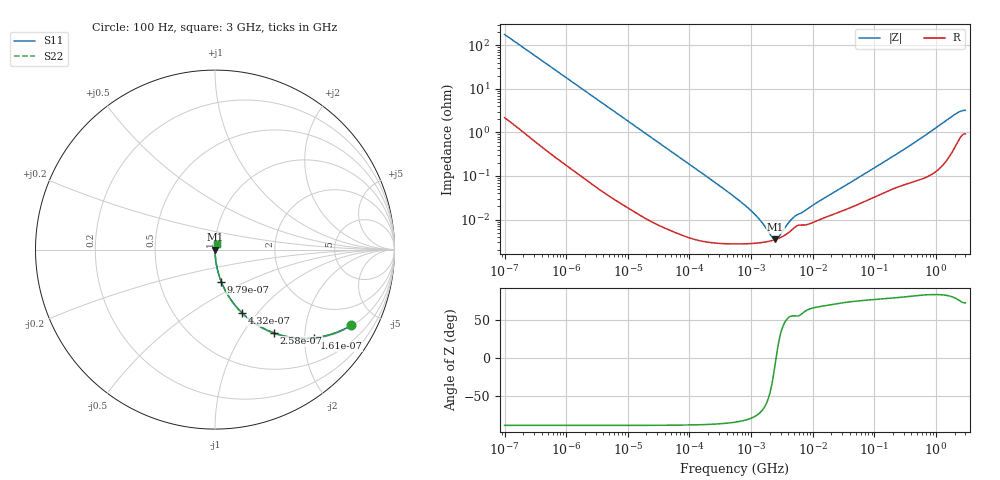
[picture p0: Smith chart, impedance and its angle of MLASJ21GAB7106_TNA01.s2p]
! MLASJ21GAB7106_TNA01  S-PARAMETER MODEL  ( Standard Model )
! Model Generated by TAIYO YUDEN Corporation (http://www.ty-top.com)
! Version 1.0
! TAIYO YUDEN Control No. 220601
! Copyright(c) 2009 TAIYO YUDEN CO.,LTD. All Rights Reserved.
! Product Description (link to TY-COMPAS)
! https://ds.yuden.co.jp/TYCOMPAS/or/detail?pn=MLASJ21GAB7106KTNA01&u=M
! Products Name : Multilayer Ceramic Capacitors
! Characteristics :
!  Capacitance : 10 [uF] , Rated Voltage : 6.3 [V] , TCC : X7R
!  Case Size : 2.0 x 1.25 / 0.079 x 0.049 [mm/inch] , Thickness : 1.25 / 0.049 [mm/inch]
!  (Conditions: Temperature = 25 [degC] , DC Bias Voltage = 0 [V])
! External Node Assignments :
!  1  o---| |---o  2
! GND o---------o GND
! Frequency Range : 100Hz  -  3GHz  [ 401 STEP ]
# MHZ S RI R 50
! Freq[MHz].  S11 Real  S11 Imag  S21 Real  S21 Imag  S12 Real  S12 Imag  S22 Real  S22 Imag
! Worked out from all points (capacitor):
!   401 points, 100 Hz to 3 GHz, reference 50 ohm
!   read as one part in series: C = 8.92 uF near 109 Hz
!   lowest |Z| = 3.49 mohm at 2.471 MHz (marker M1)
!   series resonance near 2.541 MHz, so ESL is about 440 pH
!   S11 on the Smith chart (normalised r, x): 100 Hz: 1.04, -3.56; 161 Hz: 1.03, -2.23; 258 Hz: 1.02, -1.39; 432 Hz: 1.01, -0.83; 979 Hz: 1.00, -0.37; 3 GHz: 1.02, +0.06
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0.0001  0.7575 -0.4225  0.2425 0.4225  0.2425 0.4225  0.7575 -0.4225
0.000114  0.7083 -0.4485  0.2917 0.4485  0.2917 0.4485  0.7083 -0.4485
0.000161  0.553 -0.4914  0.447 0.4914  0.447 0.4914  0.553 -0.4914
0.000258  0.3282 -0.4641  0.6718 0.4641  0.6718 0.4641  0.3282 -0.4641
0.000432  0.1505 -0.3525  0.8495 0.3525  0.8495 0.3525  0.1505 -0.3525
0.000636  0.0766 -0.2611  0.9234 0.2611  0.9234 0.2611  0.0766 -0.2611
0.000979  0.0346 -0.1781  0.9654 0.1781  0.9654 0.1781  0.0346 -0.1781
0.001788  0.0111 -0.1003  0.9889 0.1003  0.9889 0.1003  0.0111 -0.1003
0.005476  0.00143 -0.0333  0.9986 0.0333  0.9986 0.0333  0.00143 -0.0333
0.031977  0.000106 -0.00577  0.9999 0.00577  0.9999 0.00577  0.000106 -0.00577
0.547723  2.76e-05 -0.000324  1 0.000324  1 0.000324  2.76e-05 -0.000324
0.87939  2.79e-05 -0.000186  1 0.000186  1 0.000186  2.79e-05 -0.000186
1.352413  2.91e-05 -9.83e-05  1 9.83e-05  1 9.83e-05  2.91e-05 -9.83e-05
1.53882  2.98e-05 -7.62e-05  1 7.62e-05  1 7.62e-05  2.98e-05 -7.62e-05
2.470636  3.47e-05 -4.02e-06  1 4.02e-06  1 4.02e-06  3.47e-05 -4.02e-06
4.323298  5.36e-05 7.74e-05  0.9999 -7.74e-05  0.9999 -7.74e-05  5.36e-05 7.74e-05
9.794414  8.42e-05 0.000191  0.9999 -0.000191  0.9999 -0.000191  8.42e-05 0.000191
175.1444  0.000473 0.00246  0.9995 -0.00246  0.9995 -0.00246  0.000473 0.00246
513.708  0.000835 0.00661  0.9992 -0.00661  0.9992 -0.00661  0.000835 0.00661
2036.508  0.00528 0.0255  0.9947 -0.0255  0.9947 -0.0255  0.00528 0.0255
2525.516  0.00871 0.0293  0.9913 -0.0293  0.9913 -0.0293  0.00871 0.0293
3000  0.0101 0.0304  0.9899 -0.0304  0.9899 -0.0304  0.0101 0.0304
